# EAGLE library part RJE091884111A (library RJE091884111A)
Modular Jacks - Single port, 8P8C, R/A, shielded, Tab down, without LED Source: Datasheet
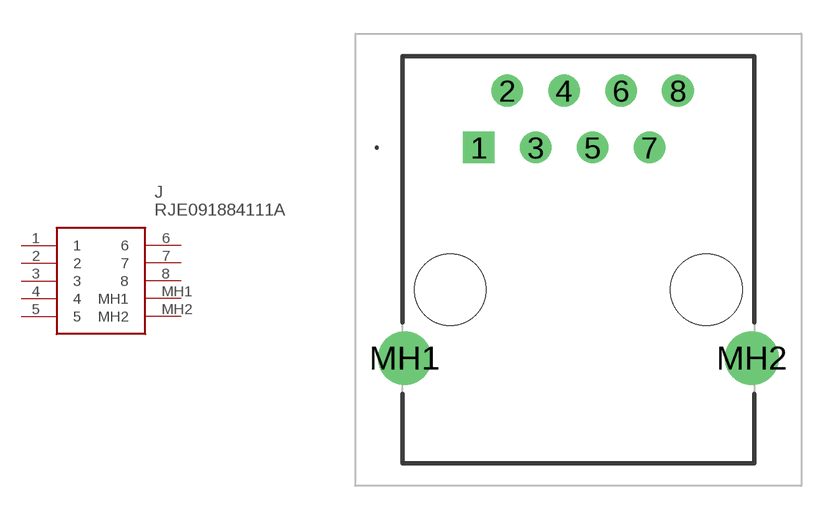
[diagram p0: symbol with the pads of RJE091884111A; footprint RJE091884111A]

Designator prefix J

## RJE091884111A (Description: Modular Jacks - Single port, 8P8C, R/A, shielded, Tab down, without LED; Height: 13.4mm; Manufacturer_Name: Amphenol Communications Solutions; Manufacturer_Part_Number: RJE091884111A)  [RJE091884111A]
1  1
2  2
3  3
4  4
5  5
6  6
7  7
8  8
MH1  MH1
MH2  MH2

## Footprint RJE091884111A (pad centres in mm)
RJE091884111A-1
drill 0.9 pad 1.4 square: 1 0,0
drill 0.9 pad 1.4: 2 1.27,2.54; 3 2.54,0; 4 3.81,2.54; 5 5.08,0; 6 6.35,2.54; 7 7.62,0; 8 8.89,2.54
drill 1.6 pad 2.4: MH1 -3.305,-9.4; MH2 12.195,-9.4
hole 3.2 at -1.27,-6.35
hole 3.2 at 10.16,-6.35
